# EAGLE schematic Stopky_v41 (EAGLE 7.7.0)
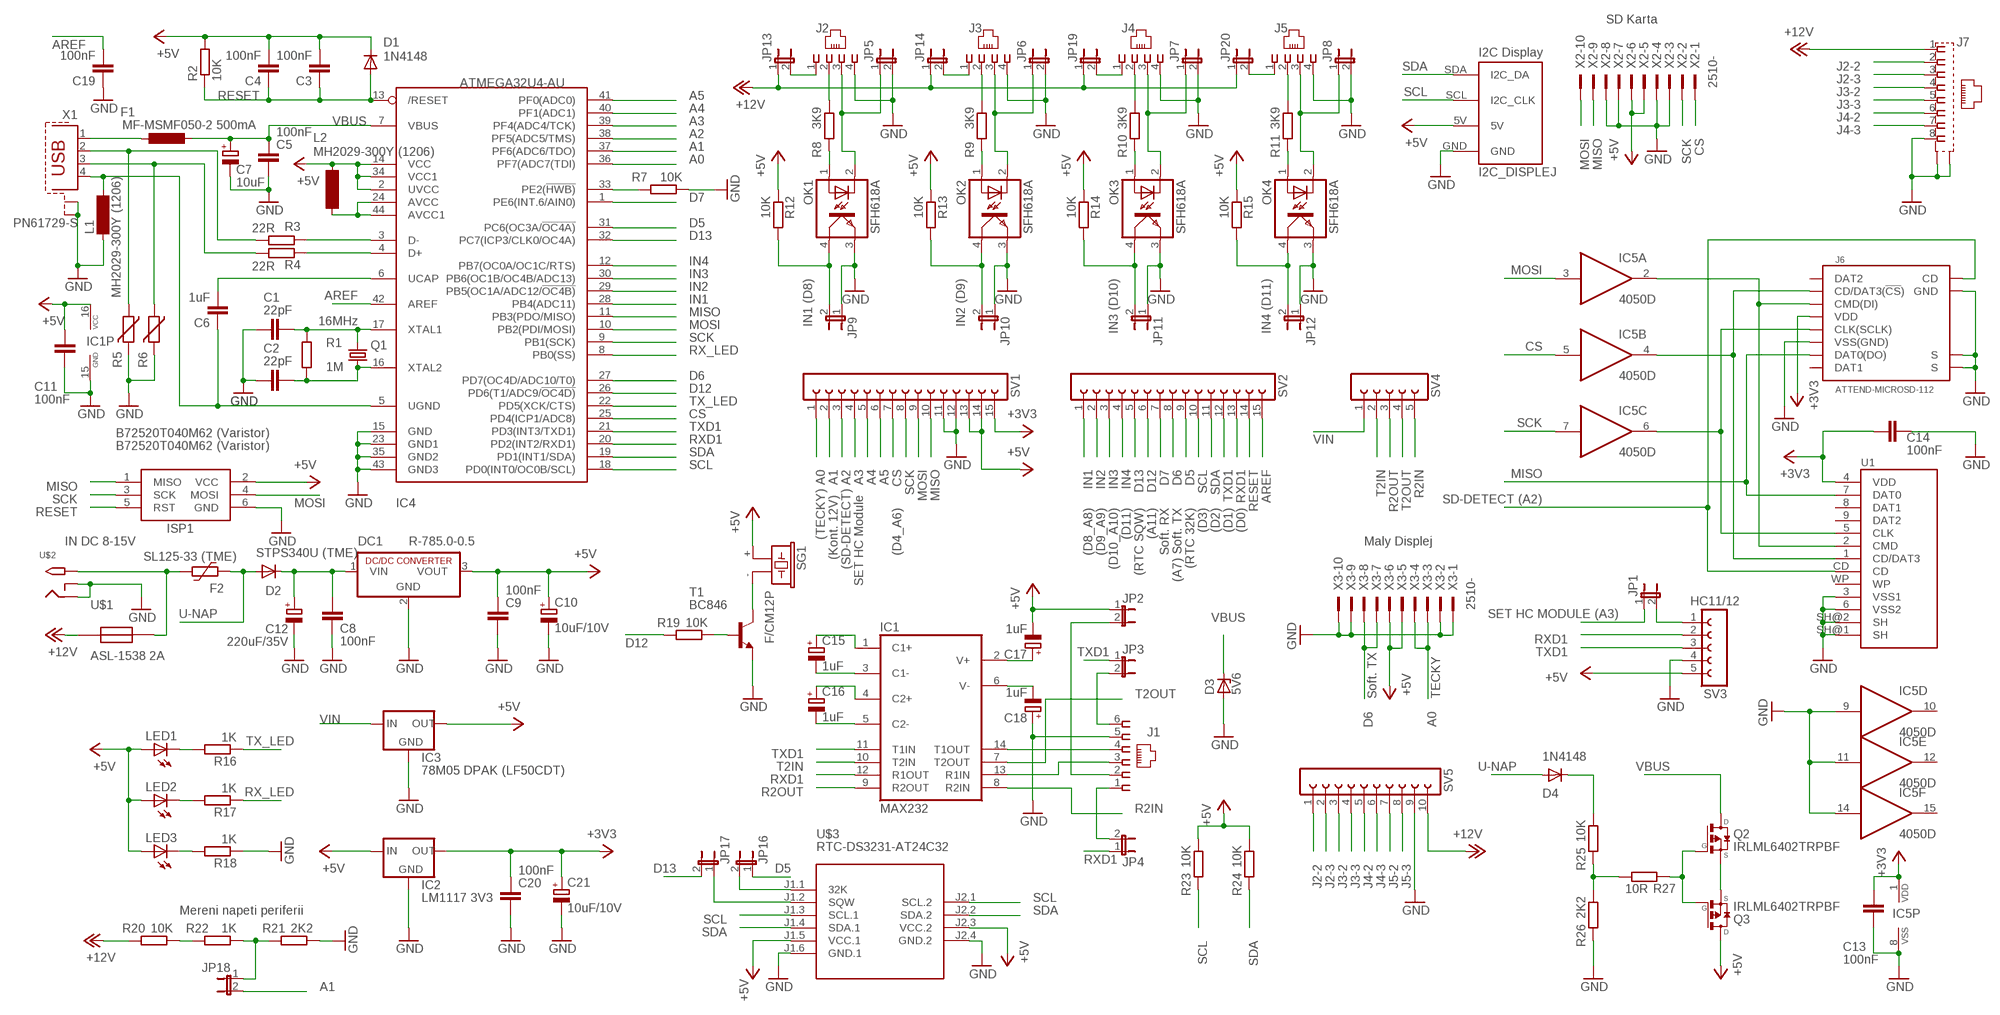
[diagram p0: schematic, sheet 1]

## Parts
C1  22pF  C-EUC1206  [C1206]
C2  22pF  C-EUC1206  [C1206]
C3  100nF  C-EUC1206  [C1206]
C4  100nF  C-EUC1206  [C1206]
C5  100nF  C-EUC1206  [C1206]
C6  1uF  C-EUC1206  [C1206]
C7  10uF  CPOL-EUSMCC  [SMC_C]
C8  100nF  C-EUC1206  [C1206]
C9  100nF  C-EUC1206  [C1206]
C10  10uF/10V  CPOL-EU153CLV-0405  [153CLV-0405]
C11  100nF  C-EUC1206  [C1206]
C12  220uF/35V  CPOL-EU153CLV-0810  [153CLV-0810]
C13  100nF  C-EUC1206  [C1206]
C14  100nF  C-EUC1206  [C1206]
C15  1uF  CPOL-EUSMCA  [SMC_A]
C16  1uF  CPOL-EUSMCA  [SMC_A]
C17  1uF  CPOL-EUSMCA  [SMC_A]
C18  1uF  CPOL-EUSMCA  [SMC_A]
C19  100nF  C-EUC1206  [C1206]
C20  100nF  C-EUC1206  [C1206]
C21  10uF/10V  CPOL-EU153CLV-0405  [153CLV-0405]
D1  1N4148  PMLL41SOD80C  [SOD80C]
D2  STPS340U (TME)  DIODE-SMB  [SMB]
D3  5V6  ZENER-DIODESOD80C  [SOD80C]
D4  1N4148  PMLL41SOD80C  [SOD80C]
DC1  R-785.0-0.5  R-78C5.0-1.0  [SIP3]
F1  MF-MSMF050-2 500mA  L-EUL1812  [L1812]
F2  SL125-33 (TME)  2920L100  [2920L]
I2C_DISPLEJ  I2C Display  I2C_HEADER5V  [I2C_HEADER_FOOTPRINT]
IC1  MAX232  MAX3232CSE  [SO16]
IC2  LM1117 3V3  LM1117  [SOT223]
IC3  78M05 DPAK (LF50CDT)  LP2950CDT-5.0  [DPACK]
IC4  ATMEGA32U4-AU  [TQFP44]
IC5  4050D  [SO16]
ISP1  AVRISP-6  [AVRISP]
J1  520250-3  [520250-3]
J2  215875-3  [215875-3]
J3  215875-3  [215875-3]
J4  215875-3  [215875-3]
J5  215875-3  [215875-3]
J6  ATTEND-MICROSD-112  [ATTEND-112]
J7  555153-1  [555153-1]
JP1  JP1E  [JP1]
JP2  JP1E  [JP1]
JP3  JP1E  [JP1]
JP4  JP1E  [JP1]
JP5  JP1E  [JP1]
JP6  JP1E  [JP1]
JP7  JP1E  [JP1]
JP8  JP1E  [JP1]
JP9  JP1E  [JP1]
JP10  JP1E  [JP1]
JP11  JP1E  [JP1]
JP12  JP1E  [JP1]
JP13  JP1E  [JP1]
JP14  JP1E  [JP1]
JP16  JP1E  [JP1]
JP17  JP1E  [JP1]
JP18  JP1E  [JP1]
JP19  JP1E  [JP1]
JP20  JP1E  [JP1]
L1  MH2029-300Y (1206)  SM-1206  [SM-1206]
L2  MH2029-300Y (1206)  SM-1206  [SM-1206]
LED1  LEDCHIPLED_1206  [CHIPLED_1206]
LED2  LEDCHIPLED_1206  [CHIPLED_1206]
LED3  LEDCHIPLED_1206  [CHIPLED_1206]
OK1  SFH618A  SFH618A-3X007  [SMD4-7]
OK2  SFH618A  SFH618A-3X007  [SMD4-7]
OK3  SFH618A  SFH618A-3X007  [SMD4-7]
OK4  SFH618A  SFH618A-3X007  [SMD4-7]
Q1  16MHz  CRYSTALSM49  [SM49]
Q2  IRLML6402TRPBF  AO3401A  [SOT23]
Q3  IRLML6402TRPBF  AO3401A  [SOT23]
R1  1M  R-EU_R1206  [R1206]
R2  10K  R-EU_R1206  [R1206]
R3  22R  R-EU_R1206  [R1206]
R4  22R  R-EU_R1206  [R1206]
R5  B72520T040M62 (Varistor)  VARISTORCN1206  [CT/CN1206]
R6  B72520T040M62 (Varistor)  VARISTORCN1206  [CT/CN1206]
R7  10K  R-EU_R1206  [R1206]
R8  3K9  R-EU_R1206  [R1206]
R9  3K9  R-EU_R1206  [R1206]
R10  3K9  R-EU_R1206  [R1206]
R11  3K9  R-EU_R1206  [R1206]
R12  10K  R-EU_R1206  [R1206]
R13  10K  R-EU_R1206  [R1206]
R14  10K  R-EU_R1206  [R1206]
R15  10K  R-EU_R1206  [R1206]
R16  1K  R-EU_R1206  [R1206]
R17  1K  R-EU_R1206  [R1206]
R18  1K  R-EU_R1206  [R1206]
R19  10K  R-EU_R1206  [R1206]
R20  10K  R-EU_R1206  [R1206]
R21  2K2  R-EU_R1206  [R1206]
R22  1K  R-EU_R1206  [R1206]
R23  10K  R-EU_R1206  [R1206]
R24  10K  R-EU_R1206  [R1206]
R25  10K  R-EU_R1206  [R1206]
R26  2K2  R-EU_R1206  [R1206]
R27  10R  R-EU_R1206  [R1206]
SG1  F/CM12P  [F/CM12P]
SV1  FE15-1  [FE15]
SV2  FE15-1  [FE15]
SV3  HC11/12  FE05-1  [FE05-1]
SV4  FE05-1  [FE05-1]
SV5  FE10-1  [FE10]
T1  BC846  [SOT23]
U1  SDCARD-SOCKET4UCON  [SDCARD-SOCKET]
U$1  ASL-1538 2A  AUTO-MALASL-1538  [SL-1538]
U$2  2.1MMJACKTHM  [PJ-102A]
U$3  RTC-DS3231-AT24C32  [RTC-DS3231-AT24C32]
X1  PN61729-S  [PN61729-S]
X2  2510-  [PAK100/2500-10]
X3  2510-  [PAK100/2500-10]

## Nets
+3V3 [3V3]: C13.2 C14.2 C20.2 C21.+ IC2.2(OUT) IC5.1(P:VDD) J6.VDD SV1.15 U1.4(VDD)
+5V [5V]: C3.2 C4.2 C9.2 C10.+ C11.2 C17.- D1.C DC1.3(VOUT) I2C_DISPLEJ.5V IC1.16(VCC) IC2.3(IN) IC3.3(OUT) IC4.2(UVCC) IC4.14(VCC) IC4.34(VCC1) ISP1.2(VCC) JP2.1 L2.2 LED1.A LED2.A LED3.A Q3.3(D) R2.2 R12.1 R13.1 R14.1 R15.1 R23.1 R24.1 SG1.+ SV1.13 SV1.14 SV3.5 U$3.J1.5(VCC.1) U$3.J2.3(VCC.2) X2.5 X2.6 X3.5 X3.6
+12V [12V]: J7.1 JP13.1 JP14.1 JP19.1 JP20.1 R20.2 SV5.10 U$1.P$1
A0: IC4.36(PF7(ADC7(TDI)) SV1.1 X3.3 X3.4
A1: IC4.37(PF6(ADC6/TDO)) JP18.2 SV1.2
A2: IC4.38(PF5(ADC5/TMS)) J6.CD SV1.3 U1.CD
A3: IC4.39(PF4(ADC4/TCK)) JP1.1 SV1.4
A4: IC4.40(PF1(ADC1)) SV1.5
A5: IC4.41(PF0(ADC0)) SV1.6
AREF: C19.2 IC4.42(AREF) SV2.15
CS: IC4.25(PD4(ICP1/ADC8)) IC5.5(B:I) SV1.7 X2.1
D5: IC4.31(PC6(OC3A/!OC4A)) JP16.1 SV2.9
D6: IC4.27(PD7(OC4D/ADC10/T0)) SV2.8 X3.7 X3.8
D7: IC4.1(PE6(INT.6/AIN0)) SV2.7
D12: IC4.26(PD6(T1/ADC9/!OC4D)) R19.2 SV2.6
D13: IC4.32(PC7(ICP3/CLK0/OC4A)) JP17.2 SV2.5
GND [GND]: C1.1 C2.1 C5.1 C7.- C8.1 C9.1 C10.- C11.1 C12.- C13.1 C14.1 C18.+ C19.1 C20.1 C21.- D3.A DC1.2(GND) I2C_DISPLEJ.GND IC1.15(GND) IC2.1(GND) IC3.4(GND) IC4.15(GND) IC4.23(GND1) IC4.35(GND2) IC4.43(GND3) IC5.8(P:VSS) IC5.9(D:I) IC5.11(E:I) IC5.14(F:I) ISP1.6(GND) J1.5 J2.4 J3.4 J4.4 J5.4 J6.GND J6.S1(S) J6.S2(S) J6.VSS(VSS(GND)) J7.8 J7.G1(S1) J7.G2(S2) JP5.2 JP6.2 JP7.2 JP8.2 JP9.1 JP10.1 JP11.1 JP12.1 L1.1 OK1.3(EMIT) OK2.3(EMIT) OK3.3(EMIT) OK4.3(EMIT) R5.2 R6.2 R7.1 R18.1 R21.1 R26.2 SV1.11 SV1.12 SV3.4 SV5.9 T1.2(E) U1.3(VSS1) U1.6(VSS2) U1.SH@1(SH) U1.SH@2(SH) U$2.RING U$2.RING_SW U$3.J1.6(GND.1) U$3.J2.4(GND.2) X1.S1 X1.S2 X2.3 X2.4 X2.7 X2.8 X3.1 X3.2 X3.9 X3.10
IN1: IC4.28(PB4(ADC11)) JP9.2 OK1.4(COL) R12.2 SV2.1
IN2: IC4.29(PB5(OC1A/ADC12/!OC4B)) JP10.2 OK2.4(COL) R13.2 SV2.2
IN3: IC4.30(PB6(OC1B/OC4B/ADC13)) JP11.2 OK3.4(COL) R14.2 SV2.3
IN4: IC4.12(PB7(OC0A/OC1C/RTS)) JP12.2 OK4.4(COL) R15.2 SV2.4
J2-2: J2.2 J7.2 R8.1 SV5.1
J2-3 [GND]: J2.3 J7.3 JP5.1 OK1.2(C) SV5.2
J3-2: J3.2 J7.4 R9.1 SV5.3
J3-3 [GND]: J3.3 J7.5 JP6.1 OK2.2(C) SV5.4
J4-2: J4.2 J7.6 R10.1 SV5.5
J4-3 [GND]: J4.3 J7.7 JP7.1 OK3.2(C) SV5.6
J5-2: J5.2 R11.1 SV5.7
J5-3 [GND]: J5.3 JP8.1 OK4.2(C) SV5.8
MISO: IC4.11(PB3(PDO/MISO)) ISP1.1(MISO) J6.DAT0(DAT0(DO)) SV1.10 U1.7(DAT0) X2.9
MOSI: IC4.10(PB2(PDI/MOSI)) IC5.3(A:I) ISP1.4(MOSI) SV1.9 X2.10
N$1 [GND]: C6.1 IC4.5(UGND) L1.2 X1.4
N$2 [USB]: F1.1 X1.1
N$3: C2.2 IC4.16(XTAL2) Q1.1 R1.1
N$4: C1.2 IC4.17(XTAL1) Q1.2 R1.2
N$5: IC4.33(PE2(!HWB)) R7.2
N$6 [5V]: IC4.24(AVCC) IC4.44(AVCC1) L2.1
N$7: R20.1 R22.2
N$8 [12V]: J3.1 JP14.2
N$9: IC4.3(D-) R3.1
N$10: IC4.4(D+) R4.1
N$11: R3.2 R5.1 X1.2
N$12: R4.2 R6.1 X1.3
N$13: C6.2 IC4.6(UCAP)
N$14: LED3.C R18.2
N$15: C17.+ IC1.2(V+)
N$16: C18.- IC1.6(V-)
N$17: C15.- IC1.3(C1-)
N$18: C16.- IC1.5(C2-)
N$19: C16.+ IC1.4(C2+)
N$20: C15.+ IC1.1(C1+)
N$21: IC1.14(T1OUT) J1.4
N$22: IC1.13(R1IN) J1.3
N$23 [5V]: J1.2 JP2.2
N$24: J1.6 JP3.2
N$25: J1.1 JP4.2
N$26 [12V]: J2.1 JP13.2
N$27 [5V]: SG1.- T1.3(C)
N$28: JP18.1 R21.2 R22.1
N$29: OK1.1(A) R8.2
N$30 [12V]: J4.1 JP19.2
N$31 [12V]: J5.1 JP20.2
N$32: OK2.1(A) R9.2
N$33 [12V]: F2.2 U$1.P$2 U$2.TIP
N$34: JP16.2 U$3.J1.1(32K)
N$35: OK3.1(A) R10.2
N$36: JP1.2 SV3.1
N$37: JP17.1 U$3.J1.2(SQW)
N$38: OK4.1(A) R11.2
N$39: R25.2 R26.1 R27.1
N$40: R19.1 T1.1(B)
N$41: IC5.2(A:O) J6.CMD(CMD(DI)) U1.2(CMD)
N$42: LED1.C R16.2
N$43: LED2.C R17.2
N$44: IC5.4(B:O) J6.DAT3(CD/DAT3(!CS!)) U1.1(CD/DAT3)
N$45: IC5.6(C:O) J6.CLK(CLK(SCLK)) U1.5(CLK)
N$46: D4.C R25.1
N$47: Q2.1(G) Q3.1(G) R27.2
N$48 [USB]: Q2.2(S) Q3.2(S)
R2IN: IC1.8(R2IN) SV4.5
R2OUT: IC1.9(R2OUT) SV4.3
RESET: C3.1 C4.1 D1.A IC4.13(/RESET) ISP1.5(RST) R2.1 SV2.14
RX_LED: IC4.8(PB0(SS)) R17.1
RXD1: IC1.12(R1OUT) IC4.20(PD2(INT2/RXD1)) JP4.1 SV2.13 SV3.2
SCK: IC4.9(PB1(SCK)) IC5.7(C:I) ISP1.3(SCK) SV1.8 X2.2
SCL: I2C_DISPLEJ.SCL(I2C_CLK) IC4.18(PD0(INT0/OC0B/SCL)) R23.2 SV2.10 U$3.J1.3(SCL.1) U$3.J2.1(SCL.2)
SDA: I2C_DISPLEJ.SDA(I2C_DA) IC4.19(PD1(INT1/SDA)) R24.2 SV2.11 U$3.J1.4(SDA.1) U$3.J2.2(SDA.2)
T2IN: IC1.10(T2IN) SV4.2
T2OUT: IC1.7(T2OUT) SV4.4
TX_LED: IC4.22(PD5(XCK/CTS)) R16.1
TXD1: IC1.11(T1IN) IC4.21(PD3(INT3/TXD1)) JP3.1 SV2.12 SV3.3
U-NAP [12V]: D2.A D4.A F2.1
VBUS [USB]: C5.2 C7.+ D3.C F1.2 IC4.7(VBUS) Q2.3(D)
VIN [12V]: C8.2 C12.+ D2.C DC1.1(VIN) IC3.1(IN) SV4.1
Unconnected: IC5.10(D:O) IC5.12(E:O) IC5.15(F:O) J6.DAT1 J6.DAT2 U1.8(DAT1) U1.9(DAT2) U1.WP

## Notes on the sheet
- SD Karta
- AREF
- SDA | J2-2
- J2-3
- SCL | J3-2
- RESET | A5 | J3-3
- A4 | J4-2
- VBUS | A3 | J4-3
- A2 | MOSI | MISO | SCK | CS
- A1
- A0
- D7
- D5
- D13
- IN4 | MOSI
- IN3 | IN1 (D8) | IN2 (D9) | IN3 (D10) | IN4 (D11)
- AREF | IN2
- IN1
- MISO
- MOSI
- SCK | CS
- RX_LED
- D6
- D12
- TX_LED
- CS | SCK
- TXD1
- RXD1 | VIN
- SDA
- SCL | (TECKY) A0 | A1 | (SD-DETECT) A2 | A3 | A4 | A5 | CS | SCK | MOSI | MISO | IN1 | IN2 | IN3 | IN4 | D13 | D12 | D7 | D6 | D5 | SCL | SDA | TXD1 | RXD1 | RESET | AREF | T2IN | R2OUT | T2OUT | R2IN | MISO
- MISO
- SCK | (Kont. 12V) | SET HC Module | SD-DETECT (A2)
- RESET | MOSI | (D4_A6) | (D8_A8) | (D9_A9) | (D10_A10) | (D11) | (RTC SQW) | (A11) | Soft. RX | (A7) Soft. TX | (RTC 32K) | (D3) | (D2) | (D1) | (D0)
- IN DC 8-15V | Maly Displej
- U-NAP | SET HC MODULE (A3)
- VBUS
- RXD1
- D12 | TXD1 | TXD1
- T2OUT | Soft. TX | TECKY
- D6 | A0
- VIN
- TX_LED
- TXD1
- T2IN | U-NAP | VBUS
- RXD1
- RX_LED | R2OUT
- R2IN
- D13 | D5 | RXD1 | J2-2 | J2-3 | J3-2 | J3-3 | J4-2 | J4-3 | J5-2 | J5-3
- SCL
- Mereni napeti periferii | SCL | SDA
- SDA
- SCL | SDA
- A1

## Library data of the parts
C1-C6 C8 C9 C11 C13 C14 C19 C20 = rcl:C-EU: CAPACITOR, European symbol
C7 C10 C12 C15-C18 C21 = rcl:CPOL-EU: POLARIZED CAPACITOR, European symbol
D1 D4 = diode:PMLL41*: High-speed diodes
D2 = diode:DIODE-: DIODE
D3 = diode:ZENER-DIODE: Z-Diode
DC1 = dc-dc-converter:R-78C*-1.0: INNOLINE DC/DC-Converter 1.0 AMP SIP3 Single Output Source: Data sheet
F1 = rcl:L-EU: INDUCTOR, European symbol
F2 = polyfuse-smd_10:?: Polyfuse Resettable PTC; MF: Littelfuse; MPN: 2920L100; OC_FARNELL: 1822225; OC_NEWARK: 18M4792
I2C_DISPLEJ = I2C_Header:I2C_HEADER
IC1 = maxim:MAX3232*: True RS-232 Transceivers 3.0V to 5.5V, Low-Power up to 1Mbps, Using Four 0.1µF External Capacitors Source: http://pdfserv.maxim-ic.com/en/ds/MAX3222-MAX3241.pdf; MPN: MAX3232CSE; OC_FARNELL: 9725490; OC_NEWARK: 90C2890
IC2 = v-reg-3:LM1117
IC3 = v-reg:LP2950?*: Source: http://cache.national.com/ds/LP/LP2950.pdf
IC4 = adafruit:ATMEGA32U4: http://www.ladyada.net/library/eagle
IC5 = 40xx:4050: Hex non-inverting BUFFER
ISP1 = adafruit:AVRISP: AVR ISP HEADER Standard 6 pin header for AVR programming
J1 = con-amp:520250-3: AMP connector
J2-J5 = con-amp:215875-3: AMP connector
J6 = sd-mmc:ATTEND-MICROSD-112: Attend microSD socket Datasheet: Attend 112 microSD socket.
J7 = con-amp:555153-1: AMP connector
JP1-JP14 JP16-JP20 = jumper:JP1E: JUMPER
L1 L2 = inductor-neosid:SM-1206: INDUCTOR; OC_FARNELL: unknown; OC_NEWARK: unknown
LED1-LED3 = led:LED: LED
OK1-OK4 = optocoupler:SFH618?*: Optocoupler, Phototransistor Output, Low Input Current Source: Data sheet; OC_FARNELL: unknown; OC_NEWARK: unknown
Q1 = crystal:CRYSTAL: CRYSTAL; OC_FARNELL: unknown; OC_NEWARK: unknown
Q2 Q3 = transistor-fet:AO3401A: P-Channel Enhancement MOSFET
R1-R4 R7-R27 = rcl:R-EU_: RESISTOR, European symbol
R5 R6 = varistor:VARISTOR: VARISTOR
SG1 = buzzer:F/CM12P: BUZZER; OC_FARNELL: unknown; OC_NEWARK: unknown
SV1 SV2 = con-lsta:FE15-1: FEMALE HEADER; OC_FARNELL: unknown; OC_NEWARK: unknown
SV3 SV4 = con-lsta:FE05-1: FEMALE HEADER; OC_FARNELL: unknown; OC_NEWARK: unknown
SV5 = con-lsta:FE10-1: FEMALE HEADER; OC_FARNELL: unknown; OC_NEWARK: unknown
T1 = transistor:BC846: NPN TRANSISTOR
U1 = Ai_Connectors:SDCARD-SOCKET: SD Memory Card Connector, push-push normal type, CD enable, WP enable
U$1 = fuse:AUTO-MALA
U$2 = adafruit:2.1MMJACK: 2.1mm x 5.5mm THM DC jack with internal switch. Digikey part #PJ-102A, 4UCON part #05537 2.1mm x 5.5mm SMT DC jack with internal switch. Digikey part #PJ-002A-SMT, 4UCON part #03267 By microbuilder.eu & adafruit.com
U$3 = diy-modules:RTC-DS3231-AT24C32: RTC Module with Battery and EEPROM based on DS3231 and AT24C32 chips Tutorial can be found here: https://edwardmallon.wordpress.com/2014/05/21/using-a-cheap-3-ds3231-rtc-at24c32-eeprom-from-ebay/ Click here to find device on ebay.com
X1 = con-berg:PN61729-S: BERG USB connector; OC_FARNELL: unknown; OC_NEWARK: unknown
X2 X3 = con-3m:2510-: 3M (TM) Pak 100 4-Wall Header Source: 3M; MF: 3M; MPN: 2510-6002UB; OC_FARNELL: 9838244; OC_NEWARK: 46F4725

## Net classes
0 default: width 0.203 mm, drill 0.406 mm, clearance 0.203 mm
1 12V: width 0.813 mm, drill 0.406 mm, clearance 0.203 mm
2 5V: width 0.61 mm, drill 0.406 mm, clearance 0.203 mm
3 GND: width 0.813 mm, drill 0.406 mm, clearance 0.203 mm
4 3V3: width 0.61 mm, drill 0.406 mm, clearance 0.203 mm
5 USB: width 0.508 mm, drill 0.406 mm, clearance 0.203 mm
